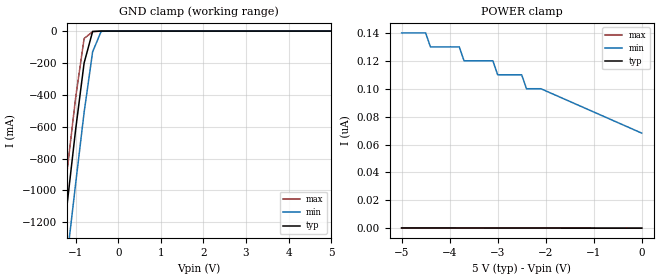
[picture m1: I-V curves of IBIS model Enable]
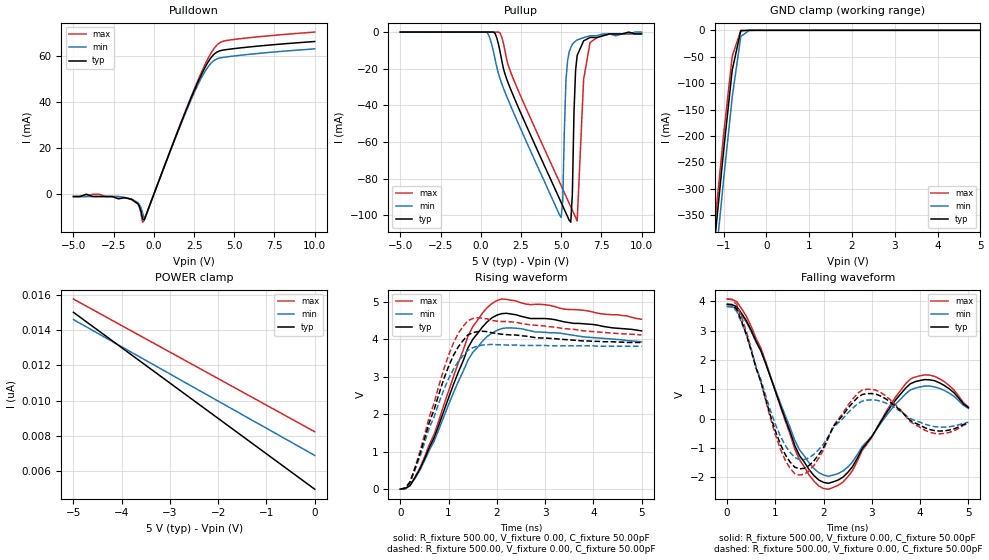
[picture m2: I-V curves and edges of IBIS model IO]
| IBIS file qs4a105.ibs
[IBIS ver]   2.1
[File name]   qs4a105.ibs
[File Rev]   1.0
[Date]   January 24, 1996
[Source]   From QSI silicon model
[Notes]   QSI provides IBIS models as a service to our customers. You
   and your company shall not distribute, convey, sell or give
   these models to anyone else without receiving prior written
   permission from QSI. QSI reserves the right to make changes to
   its products or to discontinue any semiconductor product or
   service without notice, and advises its customers to obtain
   the latest version of relevant information to verify, before
   placing orders, that the information being relied on is
   current. Please be aware that your receipt and subsequent use
   of the IBIS information provided shall serve as acceptance of
   the terms and conditions of this agreement. If you do not
   accept these terms, you should return the IBIS model and any
   other accompanying information immediately.
[Disclaimer] PLEASE BE AWARE THAT IN THE ABSENCE OF A SIGNED, WRITTEN
   AGREEMENT TO THE CONTRARY, Quality Semiconductor Incorporated
   ("QSI") IS PROVIDING THIS IBIS MODEL AS IS" AND WITHOUT AND
   WARRANTY, EXPRESSED OR IMPLIED. Further, QSI assumes no
   liability for: 1) the accuracy of the IBIS models provided to
   your company; 2) the proper functioning of these IBIS models
   in your design or for any resulting applications; or 3)
   infringement of patents, copyrights or intellectual property
   rights resulting from your use of these IBIS models. These
   commodities, technical data, and software may be U.S. export
   license controlled. As such, prior to export or re-export,
   U.S. Government approval and authorization may be required.
[Copyright]   (C) Copyright 1996 Quality Semiconductor Incorporated. All
   rights reserved. Unauthorized reproduction and/or distribution
   is strictly prohibited.
|   Component qs4a105
[Component]   qs4a105
[Manufacturer]   Quality Semiconductor Incorporated
[Package]
| Note that R_pkg is not given
| variable   typ   min   max
| Package parasitics.  Uncomment one set.
| PDIP
R_pkg   0.00   0.00   0.00
L_pkg   8.00nH   NA   NA
C_pkg   1.20pF   NA   NA
| SOIC
|R_pkg   0.00   0.00   0.00
|L_pkg   4.00nH   NA   NA
|C_pkg   0.70pF   NA   NA
| QSOP
|R_pkg   0.00   0.00   0.00
|L_pkg   2.50nH   NA   NA
|C_pkg   0.40pF   NA   NA
[Pin]  signal_name   model_name   R_pin   L_pin   C_pin
|1   E1B   Enable
2   A1   IO
3   D4   IO
4   A2   IO
5   D3   IO
6   A3   IO
7   D2   IO
8   A4   IO
9   D1   IO
10   GND   GND
11   B1   IO
12   C4   IO
13   B2   IO
14   C3   IO
15   B3   IO
16   C2   IO
17   B4   IO
18   C1   IO
|19   E2B   Enable
20   Vcc   POWER
| Models and submodels in the file (2): Enable (Input), IO (3-state)
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|   Model Enable
[Model]   Enable
Model_type   Input
Vinl =   0.00V
Vinh =   5.00V
C_comp   5.00pF   5.00pF   5.00pF
[Temperature Range]   25.00   0.12k   -40.00
[Voltage Range]   5.00V   4.50V   5.50V
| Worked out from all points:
|   GND clamp passes 1 mA (typ) near -0.49 V on its own axis
[GND_clamp]
| voltage   I(typ)   I(min)   I(max)
-5V       -10.46A    -10.75A    -10.37A
-1.4V     -1.56A     -1.9A      -1.36A
-1.2V     -1.09A     -1.42A     -880mA
-1V       -620mA     -960mA     -420mA
-800mV    -200mA     -510mA     -46.44mA
-600mV    -2.14mA    -130mA     -4.03mA
-400mV    -3.69uA    -1.72mA    -40.62uA
5V        120pA      75.77nA    120pA
[POWER_clamp]
| voltage   I(typ)   I(min)   I(max)
-5V       280pA      140nA      290pA
-4.5V     270pA      140nA      280pA
-4.4V     260pA      130nA      270pA
-3.8V     240pA      130nA      250pA
-3.7V     240pA      120nA      250pA
-3.1V     220pA      120nA      230pA
-3V       220pA      110nA      230pA
-2.5V     200pA      110nA      210pA
-2.4V     200pA      100nA      210pA
-2.1V     190pA      100nA      200pA
0V        120pA      68.19nA    130pA
|   Model IO
[Model]   IO
Model_type   3-state
Vinl =   0.00V
Vinh =   5.00V
C_comp   5.00pF   5.00pF   5.00pF
[Temperature Range]   25.00   70.00   0.00
[Voltage Range]   5.00V   4.50V   5.50V
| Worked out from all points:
|   slope of the pulldown table from 0 to 0.75 V, typ, clamps not added: 54 ohm
|   GND clamp passes 1 mA (typ) near -0.60 V on its own axis
|   rising waveform, R_fixture 500.00, V_fixture 0.00, C_fixture 50.00pF: 20-80 % time 774ps typ, 792ps min, 763ps max; typ from 0 V to 4.23 V
|   rising waveform, R_fixture 500.00, V_fixture 0.00, C_fixture 50.00pF: 20-80 % time 592ps typ, 665ps min, 563ps max; typ from 0 V to 3.92 V
|   falling waveform, R_fixture 500.00, V_fixture 0.00, C_fixture 50.00pF: 20-80 % time 525ps typ, 539ps min, 518ps max; typ from 3.89 V to 0.376 V
|   falling waveform, R_fixture 500.00, V_fixture 0.00, C_fixture 50.00pF: 20-80 % time 448ps typ, 469ps min, 443ps max; typ from 3.89 V to -0.145 V
[Pulldown]
| voltage   I(typ)   I(min)   I(max)
-5V       -1mA       -1mA       -1mA
-3.4V     -1mA       -1mA       0A
-1.4V     -2.2mA     -2.1mA     -2.1mA
-900mV    -5.3mA     -4.5mA     -5.6mA
-700mV    -10.73mA   -8.08mA    -12.14mA
-600mV    -11.18mA   -10.52mA   -11.26mA
-500mV    -9.35mA    -9.33mA    -9.38mA
2.7V      48.06mA    46.93mA    48.77mA
3.4V      57.68mA    55.57mA    59.32mA
3.9V      61.6mA     58.65mA    64.59mA
4.8V      63.03mA    59.84mA    67mA
10V       66.28mA    63.1mA     70.37mA
[Pullup]
| voltage   I(typ)   I(min)   I(max)
-5V       0A         0A         0A
400mV     0A         -287.5uA   0A
1.2V      -10.52mA   -25.42mA   -411.2uA
5V        -92.88mA   -101.1mA   -83.69mA
5.1V      -94.82mA   -92.15mA   -85.62mA
5.3V      -98.68mA   -26.3mA    -89.48mA
5.6V      -103.7mA   -8.4mA     -95.26mA
5.9V      -20.7mA    -4.9mA     -101mA
6V        -12.7mA    -4.3mA     -103mA
6.4V      -4.8mA     -3mA       -25.7mA
6.8V      -2.9mA     -2mA       -5.7mA
10V       -1mA       0A         -1mA
[GND_clamp]
| voltage   I(typ)   I(min)   I(max)
-5V       -3.69A     -3.75A     -3.67A
-1.4V     -559.6mA   -614.8mA   -529.3mA
-1.2V     -391.1mA   -446.6mA   -360.7mA
-1V       -226.9mA   -282mA     -196.7mA
-800mV    -75.3mA    -126.3mA   -49.13mA
-600mV    -834.8uA   -11.75mA   -104.4uA
-400mV    -361.2nA   -21.26uA   -22.01nA
5V        10nA       7.68nA     7.5nA
[POWER_clamp]
| voltage   I(typ)   I(min)   I(max)
-5V       15nA       14.59nA    15.75nA
-4.4V     13.8nA     13.66nA    14.85nA
-3V       11nA       11.52nA    12.75nA
0V        5nA        6.91nA     8.25nA
[Ramp]
| variable   typ   min   max
dV/dt_r   2.34/78.60p   2.29/81.25p   2.44/73.59p
dV/dt_f   2.98/50.00p   2.68/50.00p   3.28/50.00p
[Rising Waveform]
R_fixture = 500.00
V_fixture = 0.00
C_fixture = 50.00pF
L_dut = 8.00nH
C_dut = 1.20pF
| time   V(typ)   V(min)   V(max)
0s        0V         0V         0V
200ps     99.61mV    91.28mV    98.19mV
400ps     523.8mV    491.6mV    554mV
700ps     1.37V      1.28V      1.46V
1.4ns     3.77V      3.44V      4.08V
1.7ns     4.33V      3.95V      4.7V
1.9ns     4.58V      4.17V      4.96V
2.1ns     4.69V      4.29V      5.08V
2.3ns     4.68V      4.31V      5.05V
5ns       4.23V      3.94V      4.54V
[Rising Waveform]
R_fixture = 500.00
V_fixture = 0.00
C_fixture = 50.00pF
L_dut = 4.00nH
C_dut = 700.00fF
| time   V(typ)   V(min)   V(max)
0s        0V         0V         0V
200ps     188mV      171.4mV    187.6mV
400ps     911.1mV    843.3mV    974.5mV
600ps     1.78V      1.64V      1.93V
1ns       3.28V      2.95V      3.58V
1.2ns     3.8V       3.41V      4.16V
1.4ns     4.12V      3.71V      4.5V
1.6ns     4.21V      3.82V      4.58V
1.9ns     4.18V      3.87V      4.51V
5ns       3.92V      3.82V      4.12V
[Falling Waveform]
R_fixture = 500.00
V_fixture = 0.00
C_fixture = 50.00pF
L_dut = 8.00nH
C_dut = 1.20pF
| time   V(typ)   V(min)   V(max)
0s        3.89V      3.82V      4.07V
200ps     3.81V      3.74V      3.98V
400ps     3.33V      3.28V      3.48V
700ps     2.31V      2.3V       2.4V
1.5ns     -1.26V     -1.06V     -1.4V
2ns       -2.17V     -1.92V     -2.38V
2.5ns     -1.83V     -1.65V     -1.98V
3.8ns     1.19V      979.4mV    1.35V
4.3ns     1.29V      1.08V      1.44V
5ns       376.4mV    350.4mV    399.7mV
[Falling Waveform]
R_fixture = 500.00
V_fixture = 0.00
C_fixture = 50.00pF
L_dut = 4.00nH
C_dut = 700.00fF
| time   V(typ)   V(min)   V(max)
0s        3.89V      3.82V      4.07V
200ps     3.72V      3.65V      3.88V
1ns       -422.5mV   -193.5mV   -551.6mV
1.4ns     -1.65V     -1.32V     -1.87V
1.8ns     -1.43V     -1.21V     -1.59V
2.2ns     -272.6mV   -308.5mV   -257.2mV
2.8ns     821.6mV    597.9mV    971.8mV
3.2ns     756.4mV    586.3mV    873.7mV
4.2ns     -370.1mV   -237.9mV   -462.2mV
5ns       -145.3mV   -122.1mV   -160.8mV
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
